(* Logix 5000 Routine export JVL_MAC2; software revision 37.00 *)

TYPE JVL_AXIS_MAC_G3 :   // Drive Data
STRUCT
   ActualMode : DINT;   // actual Mode
   ActualPosition : REAL;   // P_IST
   ActualVelocity : REAL;   // V_IST(16)
   ActualTorque : REAL;   // ACTUAL_TORQUE
   AxisStatusError : JVL_MAC_Status_Error;   // Holds an indication of which error that is detected
   Home_Mode : DINT;   // Homemode
   RequestedMode : DINT;   // requested Mode
   RequestedPosition : REAL;   // P_SOLL
   RequestedVelocity : REAL;   // V_SOLL
   RequestedAcceleration : REAL;   // A_SOLL
   GeneralCommand : DINT;
   CommandTorque : REAL;   // Requested Torque, T_SOLL
   ZeroSearchVelocity : REAL;   // Homing velocity
   ZeroSearchPosition : REAL;   // Homing position
   ZeroSearchTorque : DINT;   // Homing torque setpoint threshold value
   ZeroSearchTThreshold : DINT;   // Threshold for torque zerosearch trigger, usually 20% lower than running torque
   TravelConst : REAL;   // Factor to multiply P_IST and P_SOLL for scaling
   VelConst : REAL;   // Factor to multiply V_SOLL and V_IST to get scaled velocity value
   HomingType : DINT;   // Holds the reqested homingtype
   LoadFactor : DINT;   // Inertia ratio motor/load
   MotorType : DINT;   // MotorType configured. 0=No Selection 1=MAC50-141-A/K (old) 2=MAC50-141-F (new), MAC400, 402, 1500, 3000, 4500 (All Encoder variations) 3=MAC800 with incremental encoder 4=MAC800 with abs. encoder
   Configured : DINT;
   MSG_OutValue : DINT;   // Used in exp. output message to the motor
   MSG_InValue : DINT;   // Used in Exp. output message, to get value from motor
   MSG_OutInstance : DINT;   // Registernumber
   MSG_InInstance : DINT;   // Registernummer
   V_SOLL_CountsPerSample : REAL;
   A_SOLL_CountsPerSample2 : REAL;
   AOI_Type : DINT;   // MAC_Disable = 1, MAC_Home = 2, MAC_Jog = 3, MAC_Position = 4, MAC_Reset = 5, MAC_Stop = 6
   Position_AppType : REAL;   // calculated Position by Application Type
   MSG_Out_Execute : BOOL;   // Enable MSG_Out
   MSG_In_Execute : BOOL;   // Enable MSG_In
   ErrorReset : BOOL;
   MSG_Out_Busy : BOOL;
   MSG_In_Busy : BOOL;
   MSG_Out_Done : BOOL;
   MSG_In_Done : BOOL;
END_STRUCT
END_TYPE

TYPE JVL_MAC_Status_Error :   // Axis Faults Status
STRUCT
   Error : BOOL;
   InitialisationError : BOOL;
   FlashMemoryError : BOOL;
   STOError : BOOL;
   NotUsed_2 : BOOL;
   NotUsed_3 : BOOL;
   OUT1 : BOOL;
   OUT2 : BOOL;
   NotUsed : BOOL;
   ControlVoltageError : BOOL;
   HomingDone : BOOL;
   MotorSupplyDetected : BOOL;
   MotorLocked : BOOL;
   CommsError : BOOL;
   CurrentLoopError : BOOL;
   ModbusSlaveError : BOOL;
   TemperatureError : BOOL;
   UndervoltageError : BOOL;
   UndervoltageDetect : BOOL;
   OvervoltageError : BOOL;
   OvercurrentError : BOOL;
   OverspeedError : BOOL;
   AllowExceedingOfSoftwareLimits : BOOL;
   EncoderError : BOOL;
   I2TError : BOOL;
   FollowingError : BOOL;
   FunctionError : BOOL;
   BreakingResistorOverTempError : BOOL;
   InPosition : BOOL;
   Accelerating : BOOL;
   Decelerating : BOOL;
   SoftwareLimitExceeded : BOOL;
END_STRUCT
END_TYPE

ADD_ON_INSTRUCTION MAC_G3_COM   (* revision 1.0 *)
VAR_IN_OUT
   JVL_IN : _03A8:MACG3Servomotor_939149E5:I:0; {required}
   JVL_OUT : _03A8:MACG3Servomotor_D07D4DE6:O:0; {required}
   MSG_IN : MESSAGE; {required}
   MSG_OUT : MESSAGE; {required}
   AXIS : JVL_AXIS_MAC_G3; {required}
END_VAR
VAR_INPUT
   ApplicationType : DINT; {required}   // Application_Type - 0=none (counts) 1=linear 2=degree
   TravelPerRev : REAL := 1.0; {required}   // Travel per Revolution. Exc. actuator w. 60mm/rev, then value=60
   GearRatio : REAL := 1.0; {required}   // Gear ratio if a gearbox is mounted. select 1 for none
   RequestedTorque : DINT := 100; {required}   // Torque in %, 0-300%
   MotorType : DINT;   // 0=MAC_G3 1=MAC50-141-A/K (old) 2=MAC50-141-F (new), MAC400, 402, 1500, 3000, 4500 (All Encoder variations) 3=MAC800 with incremental encoder 4=MAC800 with abs. encoder
END_VAR
VAR
   CountsPerRevolution : REAL; {access None}
   vel : INT; {access None}
   torque : INT; {access None}
END_VAR

ROUTINE Logic   (* structured text *)
   
   
   	//MAC050F-141F (new mini MAC), MAC400, MAC402, MAC1500-MAC4500
   	IF MotorType = 2 THEN
   	    AXIS.V_SOLL_CountsPerSample := 2.84;
   	    AXIS.A_SOLL_CountsPerSample2 := 0.003693;
   		CountsPerRevolution:= 8192.0;
   	//MAC800-MAC1200 incremental encoder
   	ELSIF MotorType = 3 THEN
   	    AXIS.V_SOLL_CountsPerSample := 2.77;
   	    AXIS.A_SOLL_CountsPerSample2 := 0.003606;
   		CountsPerRevolution:= 8000.0;
   	//MAC800-MAC1200 absolute encoder
   	ELSIF MotorType = 4 THEN
   	    AXIS.V_SOLL_CountsPerSample := 2.84;
   	    AXIS.A_SOLL_CountsPerSample2 := 0.003606;
   		CountsPerRevolution:= 8192.0;
   	//new MAC G3
   	ELSIF MotorType = 0 THEN
   	    AXIS.V_SOLL_CountsPerSample := 2.133;
   	    AXIS.A_SOLL_CountsPerSample2 := 0.002133;
   		CountsPerRevolution:= 8192.0;
   	//MAC050-141-A/K (old mini MAC)
   	ELSIF MotorType = 1 THEN
   	    AXIS.V_SOLL_CountsPerSample := 2.1;
   	    AXIS.A_SOLL_CountsPerSample2 := 0.004026;
   		CountsPerRevolution:= 4096.0;
   	ELSE
   	    AXIS.V_SOLL_CountsPerSample := 0.0;
   	    AXIS.A_SOLL_CountsPerSample2 := 0.0;
   	END_IF;
   
   	AXIS.MotorType := MotorType;
   
   	//counts
   	if ApplicationType = 0 then
   	AXIS.TravelConst := 1;
   	AXIS.VelConst:= AXIS.V_SOLL_CountsPerSample;
   	//linear
   	elsif ApplicationType = 1 then
   	AXIS.TravelConst :=(CountsPerRevolution * GearRatio) / TravelPerRev;
   	AXIS.VelConst:= AXIS.V_SOLL_CountsPerSample * 60 * GearRatio / TravelPerRev;
   	//360°
   	elsif ApplicationType = 2 then
   	AXIS.TravelConst :=(CountsPerRevolution * GearRatio) / 360;
   	AXIS.VelConst:= AXIS.V_SOLL_CountsPerSample * 60 * GearRatio / 360;
   	end_if;
   
   
   AXIS.ActualMode := JVL_IN.Operation_Mode;
   AXIS.ActualPosition := JVL_IN.Actual_Position;
   //AXIS.ActualVelocity := JVL_IN.Data[2];
   //AXIS.ActualTorque := JVL_IN.Data[3];
   vel:=JVL_IN.Actual_Velocity;
   torque:=JVL_IN.Actual_Torque;
   if MotorType=1 then
   
   AXIS.ActualVelocity := trunc(vel*7.63);
   AXIS.ActualTorque := trunc(torque * 0.293);
   else
   AXIS.ActualVelocity := trunc(vel/AXIS.VelConst);
   AXIS.ActualTorque := trunc(torque * 0.293);
   end_if;
   //AXIS.Home_Mode := JVL_IN.Data[5];
   
   AXIS.Position_AppType:= (AXIS.ActualPosition/AXIS.TravelConst);
   AXIS.AxisStatusError.Error := JVL_IN.An_Error_is_present;
   AXIS.AxisStatusError.InitialisationError := JVL_IN.Internal_Initialization_Error;
   AXIS.AxisStatusError.FlashMemoryError := JVL_IN.Flash_Memory_Error;
   AXIS.AxisStatusError.STOError := JVL_IN.STO_Circuitry_Error;
   //AXIS.AxisStatusError.NotUsed_2 := JVL_IN.Data[4].28;
   //AXIS.AxisStatusError.NotUsed_3 := JVL_IN.Data[4].29;
   //AXIS.AxisStatusError.OUT1 := JVL_IN.Data[4].30;
   //AXIS.AxisStatusError.OUT2 := JVL_IN.Data[4].31;
   //AXIS.AxisStatusError.NotUsed := JVL_IN.Data[4].16;
   AXIS.AxisStatusError.ControlVoltageError := JVL_IN.Unstable_Controlvoltage_24V;
   AXIS.AxisStatusError.HomingDone := JVL_IN.Error_And_Status.18;
   AXIS.AxisStatusError.MotorSupplyDetected := JVL_IN.AC_Voltage_Present;
   AXIS.AxisStatusError.MotorLocked := JVL_IN.PWM_Locked_Critical_Error;
   AXIS.AxisStatusError.CommsError := JVL_IN.Error_And_Status.21;
   AXIS.AxisStatusError.CurrentLoopError := JVL_IN.Error_And_Status.22;
   AXIS.AxisStatusError.ModbusSlaveError := JVL_IN.Error_And_Status.23;
   AXIS.AxisStatusError.TemperatureError := JVL_IN.Temperature_Error;
   AXIS.AxisStatusError.UndervoltageError := JVL_IN.Undervoltage_Error1;
   AXIS.AxisStatusError.UndervoltageDetect := JVL_IN.Undervoltage_Error2;
   AXIS.AxisStatusError.OvervoltageError := JVL_IN.Overvoltage_Error;
   AXIS.AxisStatusError.OvercurrentError := JVL_IN.Error_And_Status.12;
   AXIS.AxisStatusError.OverspeedError := JVL_IN.Overspeed_Error;
   AXIS.AxisStatusError.AllowExceedingOfSoftwareLimits := JVL_IN.Position_Limit_Disabled;
   AXIS.AxisStatusError.EncoderError := JVL_IN.Internal_Encoder_Error;
   AXIS.AxisStatusError.I2TError := JVL_IN.I2T_Overload_Error;
   AXIS.AxisStatusError.FollowingError := JVL_IN.Follow_Error;
   AXIS.AxisStatusError.FunctionError := JVL_IN.Function_error;
   AXIS.AxisStatusError.BreakingResistorOverTempError := JVL_IN.Error_And_Status.3;
   AXIS.AxisStatusError.InPosition := JVL_IN.In_Position;
   AXIS.AxisStatusError.Accelerating := JVL_IN.Accelerating;
   AXIS.AxisStatusError.Decelerating := JVL_IN.Decelerating;
   AXIS.AxisStatusError.SoftwareLimitExceeded := JVL_IN.Position_Limit_Error;
   
   JVL_OUT.Operation_Mode:= AXIS.RequestedMode;
   //cop(AXIS.RequestedPosition,JVL_OUT.Data[1],4);
   JVL_OUT.Requested_Position:= AXIS.RequestedPosition;
   //cop(AXIS.RequestedVelocity,JVL_OUT.Data[2],4);
   JVL_OUT.Target_Velocity:= AXIS.RequestedVelocity;
   JVL_OUT.Target_Acceleration:= AXIS.RequestedAcceleration;
   JVL_OUT.General_Command:= AXIS.GeneralCommand;
   AXIS.CommandTorque:=RequestedTorque*3.41;
   JVL_OUT.Target_Torque:=AXIS.CommandTorque;
   AXIS.MSG_Out_Done:= MSG_OUT.DN;
   AXIS.MSG_Out_Busy:= MSG_OUT.EN;
   AXIS.MSG_In_Done:= MSG_IN.DN;
   AXIS.MSG_In_Busy:= MSG_IN.EN;
   
   MSG_OUT.Instance:= AXIS.MSG_OutInstance;
   MSG_IN.Instance:= AXIS.MSG_InInstance;
   
END_ROUTINE
END_ADD_ON_INSTRUCTION

ADD_ON_INSTRUCTION MAC_G3_MAFR   (* revision 1.0, ExecuteEnableInFalse *)
VAR_IN_OUT
   AXIS : JVL_AXIS_MAC_G3; {required}
END_VAR
VAR_OUTPUT
   EN : BOOL; {access Read Only, visible}
   CommandAborted : BOOL; {access Read Only}
   DN : BOOL; {access Read Only, visible}
   ER : BOOL; {visible}
END_VAR
VAR
   State : INT; {access None}
   ExecuteStart : BOOL; {access None}
   AOI_Type : DINT; {access None}
END_VAR

ROUTINE EnableInFalse   (* structured text *)
   State := 0;
   ExecuteStart:=0;
   	//REGION STATUS SIGNALS
   
   	    DN := State = 30;
   	    CommandAborted := State = 80;
   	    EN := EnableOut;
   	    ER:= AXIS.AxisStatusError.Error;
   	//END_REGION
   
END_ROUTINE

ROUTINE Logic   (* structured text *)
   	(*********************
   		Error Reset
   	**********************)
   
   	//REGION CAPTURE EDGES
   	    if EnableIn and not ExecuteStart then
   	    	ExecuteStart:=1;
   		//elsif not EnableIn then
   			//ExecuteStart:=0;
   		end_if;
   
   	//END_REGION
   
   	//REGION STATE CHANGES
   
   	    //Re-trigger sequence from start on rising edge
   	    //Command aborted
   	    IF AXIS.AOI_Type <> AOI_Type AND
   	        State <> 0 AND
   	        State <> 90 AND
   	        State <> 30 AND
   	        State <> 80
   	    THEN
   	        State := 80;
   	    END_IF;
   
   
   	//END_REGION
   
   	//REGION STATE MACHINE
   
   	    CASE State OF
   
   	        0:
   	            IF ExecuteStart THEN
   					AOI_Type:= 5;
   					AXIS.AOI_Type:= 5;
   	                AXIS.GeneralCommand := 16#0;
   	                State := 10;
   	            END_IF;
   
   	        10:
   	            AXIS.RequestedMode := 0;
   	            AXIS.RequestedAcceleration := 0;
   	            AXIS.RequestedPosition := 0;
   	            AXIS.RequestedVelocity := 0;
   	            AXIS.GeneralCommand := 16#10000E1;
   	            IF NOT AXIS.AxisStatusError.Error and AXIS.MotorType<>1 THEN
   	                State := 20;
   
   	            END_IF;
   
   
   	        20:
   	            AXIS.GeneralCommand := 16#0;
   	            State := 30;
   
   	        30:        //reset complete, reset to idle by setting execute false
   	            ;
   
   	        80:     //Aborted by other command before completion
   	            ;
   
   	        90:       //Error while disabling, reset to idle by setting execute false
   	            ;
   
   	        ELSE
   	            ;
   
   	    END_CASE;
   
   	//END_REGION
   
   	//REGION STATUS SIGNALS
   
   	    DN := State = 30;
   	    CommandAborted := State = 80;
   	    EN := EnableOut;
   	    ER:= AXIS.AxisStatusError.Error;
   	//END_REGION
   
END_ROUTINE
END_ADD_ON_INSTRUCTION

ADD_ON_INSTRUCTION MAC_G3_MAH   (* revision 1.0, ExecuteEnableInFalse *)
VAR_IN_OUT
   Axis : JVL_AXIS_MAC_G3; {required}
END_VAR
VAR_OUTPUT
   CommandAborted : BOOL; {access Read Only}
   EN : BOOL; {access Read Only, visible}   // Enable Bit - The EN bit stays Set until the Process is Complete and the rung goes False
   DN : BOOL; {access Read Only, visible}   // Done Bit - The Done bit is Set if the Instruction Executed without Errors
   ER : BOOL; {access Read Only, visible}   // Error Bit - An Error Happened
   IP : BOOL; {access Read Only, visible}   // In Progress Bit - The In Progress bit is Set While the Axis is Moving
   PC : BOOL; {access Read Only, visible}   // Process Complete, Motion has stopped
END_VAR
VAR_INPUT
   Mode : INT; {required}   // 0 = set Encoder, 1 = Homing on Sensor, 2 = Homing on Block
   Position : REAL; {required}   // Scaled Position after setting Encoder, with Mode = 0
   Speed : REAL; {required}   // Scaled velocity
   Acceleration : REAL; {required}   // in RPM/s
   Offset : REAL; {required}   // scaled Position after Homing, with Mode = 1 or 2
   TorqueLimit : REAL; {required}   // Homing Torque in %
END_VAR
VAR
   State : INT; {access None}
   ActiveMode : INT; {access None}
   Mode0State : INT; {access None}
   Mode1State : INT; {access None}
   Mode2State : INT; {access None}
   Mode3State : INT; {access None}
   ActivePosition : DINT; {access None}
   ActiveVelocity : DINT; {access None}
   ActiveAcceleration : REAL; {access None}
   ActiveTorqueLimit : REAL; {access None}
   ExecuteStart : BOOL; {access None}
   AOI_Type : DINT; {access None}
   ActiveDeceleration : DINT; {access None}
   Ton_wait : FBD_TIMER; {access None}
   ActiveOffset : DINT; {access None}
END_VAR

ROUTINE EnableInFalse   (* structured text *)
   State := 0;
   ExecuteStart:=0;
   	//REGION STATUS SIGNALS
   
   	    DN := State = 30;
   	    CommandAborted := State = 80;
   	    ER := State = 90;
   	    IP := State <> 0 AND NOT DN AND NOT ER AND NOT CommandAborted;
   	    EN := EnableOut;
   		PC := State = 30;
   	//END_REGION
END_ROUTINE

ROUTINE Logic   (* structured text *)
   	//REGION CAPTURE EDGES
   	    if EnableIn and not ExecuteStart then
   	    	ExecuteStart:=1;
               Axis.MSG_Out_Execute := 0;
               Axis.MSG_In_Execute := 0;
   			Ton_wait.TimerEnable:=0;
   			Ton_wait.Reset:=0;
   		elsif not EnableIn then
   			ExecuteStart:=0;
   		end_if;
   
   	//END_REGION
   	//Timer
   	TONR(Ton_wait);
   
   	//REGION STATE CHANGES
   
   	    //Re-trigger sequence from start on rising edge
   
   
   	    //Command aborted
   	    IF Axis.AOI_Type <> AOI_Type AND
   	        State <> 0 AND
   	        State <> 90 AND
   	        State <> 30 AND
   	        State <> 80
   	    THEN
   	        State := 80;
   	    END_IF;
   
   
   	    //Error if motor error while executing
   	    IF Axis.AxisStatusError.Error AND
   	        State <> 0 AND
   	        State <> 90 AND
   	        State <> 30 AND
   	        State <> 80
   	    THEN
   	        State := 90;
   	    END_IF;
   	//END_REGION
   
   	//REGION STATE MACHINE
   
   
   
   	    CASE State OF
   
   	        0:
   	            //Reset static values
   	            ActiveMode := 0;
   	            ActivePosition := 0;
   	            ActiveVelocity := 0;
   				ActiveAcceleration := 0;
   	            ActiveDeceleration := 0;
   				ActiveTorqueLimit := 0;
   	            ActiveOffset := 0;
   	            //Reset mode states
   	            Mode0State := 0;
   	            Mode1State := 0;
   	            Mode2State := 0;
   	            Mode3State := 0;
   
   	            IF ExecuteStart THEN
   					//
   					AOI_Type:= 2;
   					Axis.AOI_Type:= 2;
   	                //
   					Axis.GeneralCommand := 0;
   	                ActiveMode := Mode;
   	                ActivePosition := Position * Axis.TravelConst;
   	                ActiveVelocity := (Speed) * Axis.VelConst;// * Axis.Device.Config.V_SOLL_CountsPerSample);
   	                ActiveAcceleration := ABS(Acceleration) * Axis.A_SOLL_CountsPerSample2;
   	                //set Acceleration always >=1
   	                IF ActiveAcceleration < 1 THEN
   	                    ActiveAcceleration := 1;
   	                END_IF;
   
   	                ActiveTorqueLimit := TorqueLimit * 3.41;//1024=300%;341=100%
   	                ActiveOffset := Offset * Axis.TravelConst;
   
   
   	                State := 10;
   	            END_IF;
   
   	        10:
   	            // change to velocity mode with zero setpoint to ensure motor does not run off to current position when homed
   	            IF ActiveAcceleration < 1 THEN
   	                Axis.RequestedAcceleration := 1;
   	            ELSE
   	                Axis.RequestedAcceleration := ActiveAcceleration;
   
   	            END_IF;
   	            Axis.RequestedVelocity := 0;
   	            Axis.RequestedMode := 1;
   	            // change position setpoint to new home position
   	            Axis.RequestedPosition := ActivePosition;
   	            // reset register trigger
   	            Axis.MSG_Out_Execute := 0;
   	            Axis.MSG_In_Execute := 0;
   	            // start homing
   	            State := 20;
   
   	        20:
   	            CASE ActiveMode OF
   
   	                0:  // Set Home Position
   	                    CASE Mode0State OF
   	                        0:
   	                            if Axis.MotorType=1 then
   									Axis.MSG_OutInstance := 163;
   								else
   									Axis.MSG_OutInstance := 4;
   								end_if;
   	                            Axis.MSG_OutValue:=ActivePosition;
   	                            Axis.MSG_Out_Execute := 1;
   	                            Axis.GeneralCommand := 16#0;
   	                            IF Axis.MSG_Out_Busy AND NOT Axis.MSG_Out_Done THEN
   	                                Mode0State := 10;
   	                            END_IF;
   	                        10:
   	                            IF Axis.MSG_Out_Done THEN
   	                                Axis.MSG_Out_Execute := 0;
   	                                Mode0State := 20;
   	                            END_IF;
   	                        20:
   	                            Axis.GeneralCommand := 16#10000F7;
   	                            IF ABS(Axis.ActualPosition - ActivePosition) < 50.0 THEN
   	                                Mode0State := 30;
   	                            END_IF;
   	                        30:
   	                            Axis.GeneralCommand := 16#0;
   	                            Mode0State := 50;
   	                        50:
   	                            State := 30;
   	                        ELSE
   	                            State := 90;
   	                    END_CASE;
   
   	                1:  // Home to Sensor (type 2, bidirectional)
   	                    CASE Mode1State OF
   	                       0:
   	                            // reset hominging done bit old MAC050-141A/K
   	                                IF Axis.MotorType <> 1 THEN
   	                                    Mode1State := 10;
   	                                ELSE
   		                            Axis.MSG_OutInstance := 168;
   		                            Axis.MSG_OutValue := 0;
   		                            Axis.MSG_Out_Execute := 1;
   			                            IF Axis.MSG_Out_Busy THEN
   			                                Mode1State := 5;
   			                            END_IF;
   	                                END_IF;
   	                        5:
   	                            //Ton_Wait(IN := Reg.Done,PT := t#1s);
   	                            IF Axis.MSG_Out_Done THEN
   	                                Axis.MSG_Out_Execute := 0;
   	                                Mode1State := 10;
   	                            END_IF;
   	                       10:
   	                            //Home to Sensor (type 2);set homemode=3584
   	                            Axis.MSG_OutInstance := 42;
   	                            Axis.MSG_OutValue:=3584;
   
   	                            Axis.MSG_Out_Execute := 1;
   	                            IF Axis.MSG_Out_Busy THEN
   	                                Mode1State := 15;
   	                            END_IF;
   	                       15:
   	                            IF Axis.MSG_Out_Done THEN
   	                                Axis.MSG_Out_Execute := 0;
   	                                Mode1State := 20;
   									Axis.AxisStatusError.HomingDone:=0;
   	                            END_IF;
   
   	                       20:
   	                            // set home position offset move distance
   	                            Axis.MSG_OutInstance := 38;
   	                            Axis.MSG_OutValue:=ActiveOffset;
   	                            Axis.MSG_Out_Execute := 1;
   	                            IF Axis.MSG_Out_Busy THEN
   	                                Mode1State := 30;
   	                            END_IF;
   	                        30:
   	                            IF Axis.MSG_Out_Done THEN
   	                                Axis.MSG_Out_Execute := 0;
   	                                Mode1State := 40;
   	                            END_IF;
   	                        40:
   	                            // set homing approach velocity
   	                            Axis.MSG_OutInstance := 40;
   	                            Axis.MSG_OutValue:=ActiveVelocity;// * Axis.Device.Config.V_SOLL_CountsPerSample
   	                            Axis.MSG_Out_Execute := 1;
   	                            IF Axis.MSG_Out_Busy THEN
   	                                Mode1State := 50;
   	                            END_IF;
   	                        50:
   	                            IF Axis.MSG_Out_Done THEN
   	                                Axis.MSG_Out_Execute := 0;
   	                                Mode1State := 60;
   	                            END_IF;
   	                        60:
   	                            // start homing mode
   	                            Axis.RequestedMode := 14;
   								if Axis.MotorType=1 then
   									Axis.RequestedVelocity := ActiveVelocity;
   								end_if;
   	                            if Axis.ActualMode=14 then
   	                            	Mode1State := 70;
   	                            end_if;
   	                        70:
   	                            IF Axis.AxisStatusError.HomingDone AND Axis.MotorType <> 1 THEN
   	                                Axis.RequestedVelocity := 0;
   	                                Axis.RequestedMode := 2;
   	                                Mode1State := 80;
   	                            ELSIF Axis.Home_Mode > 0 AND Axis.MotorType = 1 THEN
   	                                Axis.RequestedVelocity := 0;
   	                                Axis.RequestedMode := 2;
   	                                Mode1State := 80;
   	                            END_IF;
   	                        80:
   	                            State := 30;
   	                        ELSE
   	                            State := 90;
   	                    END_CASE;
   
   	                2:  // Home to Endstop (torque limit)
   	                    CASE Mode2State OF
   	                        0:
   	                            //Home to Endstop (torque limit);set homemode=3072
   								Axis.MSG_OutInstance := 42;
   	                            Axis.MSG_OutValue := 3072;
   	                            Axis.MSG_Out_Execute := 1;
   
   	                            IF Axis.MSG_Out_Busy THEN
   	                                Mode2State := 5;
   	                            END_IF;
   	                        5:
   	                            IF Axis.MSG_Out_Done THEN
   	                                Axis.MSG_Out_Execute := 0;
   	                                Mode2State := 10;
   	                            END_IF;
   	                        10:
   								Axis.MSG_OutInstance := 38;
   	                            Axis.MSG_OutValue := ActiveOffset;
   	                            Axis.MSG_Out_Execute := 1;
   
   	                            IF Axis.MSG_Out_Busy THEN
   	                                Mode2State := 15;
   	                            END_IF;
   	                        15:
   	                            IF Axis.MSG_Out_Done THEN
   	                                Axis.MSG_Out_Execute := 0;
   	                                Mode2State := 20;
   									Axis.AxisStatusError.HomingDone:=0;
   	                            END_IF;
   	                        20:
   								Axis.MSG_OutInstance := 40;
   	                            Axis.MSG_OutValue := ActiveVelocity;// * Axis.Device.Config.V_SOLL_CountsPerSample;
   	                            Axis.MSG_Out_Execute := 1;
   	                            IF Axis.MSG_Out_Busy THEN
   	                                Mode2State := 25;
   	                            END_IF;
   	                        25:
   	                            IF Axis.MSG_Out_Done THEN
   	                                Axis.MSG_Out_Execute := 0;
   	                                IF Axis.MotorType <> 1 THEN
   	                                    Mode2State := 34;
   	                                ELSE
   	                                    Mode2State := 30;
   	                                END_IF;
   	                            END_IF;
   	                        30:
   	                            // reset hominging done bit old MAC050-141A/K
   								Axis.MSG_OutInstance := 168;
   	                            Axis.MSG_OutValue := 0;
   	                            Axis.MSG_Out_Execute := 1;
   
   	                            IF Axis.MSG_Out_Busy THEN
   	                                Mode2State := 32;
   	                            END_IF;
   	                        32:
   
   	                            IF Axis.MSG_Out_Done THEN
   	                                Axis.MSG_Out_Execute := 0;
   	                                Mode2State := 34;
   	                            END_IF;
   	                        34:
   								Axis.MSG_OutInstance := 41;
   	                            Axis.MSG_OutValue := ActiveTorqueLimit;
   	                            Axis.MSG_Out_Execute := 1;
   
   	                            IF Axis.MSG_Out_Busy THEN
   	                                Mode2State := 37;
   	                            END_IF;
   	                        37:
   	                            IF Axis.MSG_Out_Done THEN
   	                                Axis.MSG_Out_Execute := 0;
   	                                Mode2State := 40;
   	                            END_IF;
   	                        40:
   	                            Axis.RequestedMode := 12;
   	                            // homing done-register 42 Homemode bit 16
   								if Axis.MotorType=1 then
   									Axis.RequestedVelocity := ActiveVelocity;
   								end_if;
   	                            if Axis.ActualMode=12 then
   	                            	Mode2State := 45;
   	                            end_if;
   
   	                        45:
   	                            IF Axis.AxisStatusError.HomingDone AND Axis.MotorType <> 1 THEN
   	                                Axis.RequestedVelocity := 0;
   	                                Axis.RequestedMode := 2;
   	                                Mode2State := 60;
   	                            ELSIF Axis.Home_Mode > 0 AND Axis.MotorType = 1 THEN
   	                                Axis.RequestedVelocity := 0;
   	                                Axis.RequestedMode := 2;
   	                                Mode2State := 60;
   	                            END_IF;
   
   	                        60:
   	                            State := 30;
   	                        ELSE
   	                            State := 90;
   	                    END_CASE;
   
   
   
   	            END_CASE;
   
   	        30:        //Home complete, reset to idle by setting execute false
   	            ;
   
   	        80:     //Aborted by other command before completion
   	            ;
   
   	        90:       //Error while disabling, reset to idle by setting execute false
   	            ;
   
   	        ELSE
   	            ;
   
   	    END_CASE;
   
   	//END_REGION
   
   	//REGION STATUS SIGNALS
   
   	    DN := State = 30;
   	    CommandAborted := State = 80;
   	    ER := State = 90;
   	    IP := State <> 0 AND NOT DN AND NOT ER AND NOT CommandAborted;
   	    EN := EnableOut;
   		PC := State = 30;
   	//END_REGION
END_ROUTINE
END_ADD_ON_INSTRUCTION

ADD_ON_INSTRUCTION MAC_G3_MAJ   (* revision 1.0, ExecuteEnableInFalse *)
VAR_IN_OUT
   AXIS : JVL_AXIS_MAC_G3; {required}
END_VAR
VAR_INPUT
   Direction : DINT; {required}   // 0 = CW rotation, 1 = CCW rotation
   Speed : REAL; {required}   // scaled velocity
   Acceleration : REAL := 5000.0; {required}   // in rpm/s
END_VAR
VAR_OUTPUT
   EN : BOOL; {access Read Only, visible}   // Enable Bit - The EN bit stays Set until the Process is Complete and the rung goes False
   DN : BOOL; {access Read Only, visible}   // Done Bit - The Done bit is Set if the Instruction Executed without Errors
   ER : BOOL; {access Read Only, visible}   // Error Bit - An Error Happened
   IP : BOOL; {access Read Only, visible}   // In Progress Bit - The In Progress bit is Set While the Axis is Moving
END_VAR
VAR
   ForwardStart : BOOL; {access None}
   BackwardStart : BOOL; {access None}
   State : INT; {access None}
   ActiveVelocity : REAL; {access None}
   ActiveAcceleration : REAL; {access None}
   AOI_Type : DINT; {access None}
   ActiveDeceleration : REAL; {access None}
END_VAR

ROUTINE EnableInFalse   (* structured text *)
   	//REGION CAPTURE EDGES
   	    if Direction = 0 and EnableIn then
   	    	ForwardStart:=1;
   	    elsif Direction = 1 and EnableIn then
   	    	BackwardStart:=1;
   		elsif not EnableIn then
   	    	ForwardStart:=0;
   	    	BackwardStart:=0;
   		end_if;
   
   	//END_REGION
   
   	//REGION STATE CHANGES
   
   	    //Re-trigger sequence from start on rising edge
   	    //Command aborted
   	    IF AXIS.AOI_Type <> AOI_Type AND
   	        State <> 0 AND
   	        State <> 90 AND
   	        State <> 80
   	    THEN
   	        State := 80;
   	    END_IF;
   
   
   
   	    //Error if motor error while executing
   	    IF AXIS.AxisStatusError.Error AND
   	        State <> 0 AND
   	        State <> 90 AND
   	        State <> 80
   	    THEN
   	        State := 90;
   	    END_IF;
   
   	//END_REGION
   
   	//REGION STATE MACHINE
   
   	    CASE State OF
   
   	        0:
   	            ActiveVelocity := 0;
   	            ActiveAcceleration := 0;
   	            ActiveDeceleration := 0;
   
   	            IF ForwardStart OR BackwardStart THEN
   					DN := 0;
   					AOI_Type:= 3;
   					AXIS.AOI_Type:= 3;
   	                AXIS.RequestedMode:= 1;
   	                ActiveAcceleration := ABS(Acceleration);
   
   	                //set Acceleration always >=1
   	                IF ActiveAcceleration < 1 THEN
   	                    ActiveAcceleration := 1;
   	                END_IF;
   	                IF Direction = 0 THEN
   	                    ActiveVelocity := ABS(Speed) * AXIS.VelConst;// * Axis.Device.Config.V_SOLL_CountsPerSample));
   	                    State := 10;
   	                ELSIF Direction = 1 THEN
   	                    ActiveVelocity := -1.0 * ABS(Speed)* AXIS.VelConst;// * Axis.Device.Config.V_SOLL_CountsPerSample));
   	                    State := 10;
   	                ELSE
   	                    State := 30;
   	                END_IF;
   
   	                State := 10;
   	            END_IF;
   
   	        10:
   	            IF AXIS.ActualMode = 1 THEN
   
   	                AXIS.RequestedAcceleration := ActiveAcceleration;
   	                AXIS.RequestedVelocity := ActiveVelocity;
                       State := 30;
   
   	            END_IF;
   
   	        20:
   	            IF AXIS.ActualMode = 1 THEN
   
   	                IF not EnableIn THEN
   	                    State := 30;
   	                END_IF;
   
   	            ELSE
   	                State := 80;
   	            END_IF;
   
   
   	        30:
   	            AXIS.RequestedMode := 1;
   	            AXIS.RequestedVelocity := 0;
   
   	            State := 40;
   
   	        40:
   	            IF AXIS.ActualMode = 1  THEN
   
   	                //If no motion then stop is complete
   	                IF ABS((AXIS.ActualVelocity)) <= 10.0 AND
   	                    NOT AXIS.AxisStatusError.Accelerating AND
   	                    NOT AXIS.AxisStatusError.Decelerating THEN
   	                    State := 0;
   						DN := 1;
   	                END_IF;
   
   	            ELSE
   	                State := 80;
   	            END_IF;
   
   	        80:     //Aborted by other command before completion
   	            IF NOT EnableIn THEN
   	                State := 0;
   	            END_IF;
   
   	        90:       //Error while jogging, reset to idle by setting jog inputs false
   	            IF NOT EnableIn THEN
   	                State := 0;
   	            END_IF;
   
   	        ELSE
   	            State := 90;
   
   	    END_CASE;
   
   	//END_REGION
   
   	//REGION STATUS SIGNALS
   
   	    EN:=EnableOut;
   						//(State=20 or State = 25) AND
   	                    //  AXIS.AxisStatus.AtVelocity AND
   	                    //  NOT AXIS.AxisStatus.Accelerating AND
   	                    //  NOT AXIS.AxisStatus.Decelerating;
   	    DN := State = 40;
   	    ER := State = 90;
   	    IP := State <> 0 AND NOT ER AND NOT DN;
   
   	//END_REGION
   
END_ROUTINE

ROUTINE Logic   (* structured text *)
   	//REGION CAPTURE EDGES
   	    if Direction = 0 and EnableIn then
   	    	ForwardStart:=1;
   	    elsif Direction = 1 and EnableIn then
   	    	BackwardStart:=1;
   		elsif not EnableIn then
   	    	ForwardStart:=0;
   	    	BackwardStart:=0;
   		end_if;
   
   	//END_REGION
   
   	//REGION STATE CHANGES
   
   	    //Re-trigger sequence from start on rising edge
   	    //Command aborted
   	    IF AXIS.AOI_Type <> AOI_Type AND
   	        State <> 0 AND
   	        State <> 90 AND
   	        State <> 80
   	    THEN
   	        State := 80;
   	    END_IF;
   
   
   
   	    //Error if motor error while executing
   	    IF AXIS.AxisStatusError.Error AND
   	        State <> 0 AND
   	        State <> 90 AND
   	        State <> 80
   	    THEN
   	        State := 90;
   	    END_IF;
   
   	//END_REGION
   
   	//REGION STATE MACHINE
   
   	    CASE State OF
   
   	        0:
   	            ActiveVelocity := 0;
   	            ActiveAcceleration := 0;
   	            ActiveDeceleration := 0;
   
   	            IF ForwardStart OR BackwardStart THEN
   					DN := 0;
   					AOI_Type:= 3;
   					AXIS.AOI_Type:= 3;
   	                AXIS.RequestedMode:= 1;
   	                ActiveAcceleration := ABS(Acceleration)* AXIS.A_SOLL_CountsPerSample2;
   	                //set Acceleration always >=1
   	                IF ActiveAcceleration < 1 THEN
   	                    ActiveAcceleration := 1;
   	                END_IF;
   	                IF Direction = 0 THEN
   	                    ActiveVelocity := ABS(Speed) * AXIS.VelConst;// * Axis.Device.Config.V_SOLL_CountsPerSample));
   	                    State := 10;
   	                ELSIF Direction = 1 THEN
   	                    ActiveVelocity := -1.0 * ABS(Speed)* AXIS.VelConst;// * Axis.Device.Config.V_SOLL_CountsPerSample));
   	                    State := 10;
   	                ELSE
   	                    State := 30;
   	                END_IF;
   
   	                State := 10;
   	            END_IF;
   
   	        10:
   	            IF AXIS.ActualMode = 1 THEN
   
   	                AXIS.RequestedAcceleration := ActiveAcceleration;
   	                AXIS.RequestedVelocity := ActiveVelocity;
   	                IF not EnableIn THEN
   	                    State := 30;
   	                END_IF;
   
   	            END_IF;
   
   	        20:
   	            IF AXIS.ActualMode = 1 THEN
   
   	                IF not EnableIn THEN
   	                    State := 30;
   	                END_IF;
   
   	            ELSE
   	                State := 80;
   	            END_IF;
   
   
   	        30:
   	            AXIS.RequestedMode := 1;
   	            AXIS.RequestedVelocity := 0;
   
   	            State := 40;
   
   	        40:
   	            IF AXIS.ActualMode = 1  THEN
   
   	                //If no motion then stop is complete
   	                IF ABS((AXIS.ActualVelocity)) <= 10.0 AND
   	                    NOT AXIS.AxisStatusError.Accelerating AND
   	                    NOT AXIS.AxisStatusError.Decelerating THEN
   	                    State := 0;
   						DN := 1;
   	                END_IF;
   
   	            ELSE
   	                State := 80;
   	            END_IF;
   
   	        80:     //Aborted by other command before completion
   	            IF NOT EnableIn THEN
   	                State := 0;
   	            END_IF;
   
   	        90:       //Error while jogging, reset to idle by setting jog inputs false
   	            IF NOT EnableIn THEN
   	                State := 0;
   	            END_IF;
   
   	        ELSE
   	            State := 90;
   
   	    END_CASE;
   
   	//END_REGION
   
   	//REGION STATUS SIGNALS
   
   	    EN:=EnableOut;
   						//(State=20 or State = 25) AND
   	                    //  AXIS.AxisStatus.AtVelocity AND
   	                    //  NOT AXIS.AxisStatus.Accelerating AND
   	                    //  NOT AXIS.AxisStatus.Decelerating;
   	    DN := State = 40;
   	    ER := State = 90;
   	    IP := State <> 0 AND NOT ER AND NOT DN;
   
   	//END_REGION
   
END_ROUTINE
END_ADD_ON_INSTRUCTION

ADD_ON_INSTRUCTION MAC_G3_MAM   (* revision 1.0, ExecuteEnableInFalse *)
VAR_IN_OUT
   Axis : JVL_AXIS_MAC_G3; {required}
END_VAR
VAR_INPUT
   MoveType : DINT; {required}   // 0=absolute, 1= relative
   Position : REAL; {required}   // scaled Position
   Speed : REAL; {required}   // scaled velocity
   Acceleration : REAL; {required}   // in rpm/s
END_VAR
VAR_OUTPUT
   CommandAborted : BOOL; {access Read Only}
   EN : BOOL; {visible}   // Enable Bit - The EN bit stays Set until the Process is Complete and the rung goes False
   DN : BOOL; {access Read Only, visible}   // Done Bit - The Done bit is Set if the Instruction Executed without Errors
   ER : BOOL; {access Read Only, visible}   // Error Bit - An Error Happened
   IP : BOOL; {access Read Only, visible}   // In Progress Bit - The In Progress bit is Set While the Axis is Moving
   PC : BOOL; {visible}   // Process Complete, Motion has stopped
END_VAR
VAR
   State : INT; {access None}
   ExecuteStart : BOOL; {access None}
   ActiveAbsolute : BOOL; {access None}
   ActiveVelocity : DINT; {access None}
   ActiveAcceleration : REAL; {access None}
   ActiveTargetPosition : DINT; {access None}
   StartPosition : REAL; {access None}
   AOI_Type : DINT; {access None}
END_VAR

ROUTINE EnableInFalse   (* structured text *)
   State := 0;
   ExecuteStart:=0;
   	    DN := State = 30 OR State = 35;
   		PC:= State = 30 OR State = 35;
   	    CommandAborted := State = 80;
   	    ER := State = 90;
   	    IP := State <> 0 AND NOT DN AND NOT ER AND NOT CommandAborted;
   	    EN:= EnableOut;
   
END_ROUTINE

ROUTINE Logic   (* structured text *)
   	//REGION CAPTURE EDGES
   	    if EnableIn and not ExecuteStart then
   	    	ExecuteStart:=1;
   			State:= 0;
   
   		end_if;
   
   	//END_REGION
   
   	//REGION STATE CHANGES
   
   	    //Re-trigger sequence from start on rising edge
   
   
   	    //Command aborted
   	    IF Axis.AOI_Type <> AOI_Type AND
   	        State <> 0 AND
   	        State <> 90 AND
   	        State <> 30 AND
   	        State <> 80
   	    THEN
   	        State := 80;
   	    END_IF;
   
   
   	    //Error if motor error while executing
   	    IF Axis.AxisStatusError.Error AND
   	        State <> 0 AND
   	        State <> 90 AND
   	        State <> 30 AND
   	        State <> 80
   	    THEN
   	        State := 90;
   	    END_IF;
   	//END_REGION
   
   	//REGION STATE MACHINE
   
   	    CASE State OF
   
   	        0:
   	            ActiveVelocity := 0;
   	            ActiveAcceleration := 0;
   				ActiveAbsolute := 0;
   	            ActiveTargetPosition := 0;
   
   	            IF ExecuteStart THEN
   					AOI_Type:= 4;
   					Axis.AOI_Type:= 4;
   	                Axis.RequestedMode := 2;
   	                StartPosition := Axis.ActualPosition;// *Axis.TravelConst;
   	                ActiveVelocity := ABS(Speed) * Axis.VelConst;// * Axis.Device.Config.V_SOLL_CountsPerSample);
   	                ActiveAcceleration := ABS(Acceleration)* Axis.A_SOLL_CountsPerSample2;
   	                //set Acceleration always >=1
   	                IF ActiveAcceleration < 1.0 THEN
   	                    ActiveAcceleration := 1.0;
   	                END_IF;
   
   					if MoveType= 0 then
   	                	ActiveAbsolute := 1;
   					elsif MoveType = 1 then
   						ActiveAbsolute:= 0;
   					end_if;
   
   
   
   	                IF ActiveAbsolute THEN
   	                    ActiveTargetPosition := Position *Axis.TravelConst;
   	                ELSE
   	                    ActiveTargetPosition := Position *Axis.TravelConst+ StartPosition;
   	                END_IF;
   
   	                State := 10;
   	            END_IF;
   
   	        10:
   	            IF Axis.ActualMode = 2 THEN
   	                Axis.RequestedAcceleration := ActiveAcceleration;
   	                Axis.RequestedPosition := ActiveTargetPosition;
   	                Axis.RequestedVelocity := ActiveVelocity;
   
   					State := 20;
   					(*
   	                IF ContinuousUpdate THEN
   	                    State := 25;
   	                ELSE
   	                    State := 20;
   	                END_IF;
   	                *)
   	            END_IF;
   
   	        20:
   	            IF Axis.ActualMode = 2 AND
   	                Axis.RequestedPosition = ActiveTargetPosition AND
   	                Axis.RequestedVelocity = ActiveVelocity THEN
   
   	                //If taget reached then move is complete
   	                IF ABS(ActiveTargetPosition - Axis.ActualPosition) <= 10 AND
   	                    Axis.AxisStatusError.InPosition AND
   	                    NOT Axis.AxisStatusError.Accelerating AND
   	                    NOT Axis.AxisStatusError.Decelerating THEN
   	                    State := 30;
   	                END_IF;
   
   	            ELSE
   	                State := 80;
   	            END_IF;
   
   	        30:
   	            ;
   	        (*
   	        25:
   	            IF Axis.Telegram.Input.OperatingMode = 2 AND
   	                Axis.Telegram.Output.VelocitySetpoint = DINT_TO_DWORD(ActiveVelocity) AND
   	                Axis.Telegram.Output.PositionSetpoint = DINT_TO_DWORD(ActiveTargetPosition) THEN
   
   	                IF Execute THEN
   
   	                    ActiveVelocity := LREAL_TO_DINT(ABS(Velocity) * Axis.Device.Config.V_SOLL_CountsPerSample);
   	                    ActiveAcceleration := LREAL_TO_DINT(ABS(Acceleration) * Axis.Device.Config.A_SOLL_CountsPerSample2);
   	                    //set Acceleration always >=1
   	                    IF ActiveAcceleration < 1 THEN
   	                        ActiveAcceleration := 1;
   	                    END_IF;
   	                    IF ActiveAbsolute THEN
   	                        ActiveTargetPosition := Position;
   	                    ELSE
   	                        ActiveTargetPosition := Position + StartPosition;
   	                    END_IF;
   
   	                    Axis.Telegram.Output.AccelerationSetpoint := ActiveAcceleration;
   	                    Axis.Telegram.Output.PositionSetpoint := ActiveTargetPosition;
   	                    Axis.Telegram.Output.VelocitySetpoint := ActiveVelocity;
   
   	                    //If taget reached then move is complete
   	                    IF ABS(DINT_TO_LREAL(ActiveTargetPosition - Axis.Telegram.Input.ActualPosition)) <= 5.0 AND
   	                        Axis.Telegram.Input.StatusError.InPosition AND
   	                        NOT Axis.Telegram.Input.StatusError.Accelerating AND
   	                        NOT Axis.Telegram.Input.StatusError.Decelerating THEN
   	                        State := 35;
   	                    END_IF;
   
   	                ELSE
   	                    State := 20;
   	                END_IF;
   
   	            ELSE
   	                State := 80;
   	            END_IF;
   
   	        35:
   	            IF Execute THEN
   
   	                IF ActiveAbsolute THEN
   	                    IF ActiveTargetPosition <> Position THEN
   	                        State := 20;
   	                    END_IF;
   	                ELSE
   	                    IF ActiveTargetPosition <> (Position + StartPosition) THEN
   	                        State := 25;
   	                    END_IF;
   	                END_IF;
   
   	            ELSE
   	                State := 0;
   	            END_IF;
   	        *)
   	        80:     //Aborted by other command before completion
   	           ;
   
   	        90:       //Error, reset to idle by setting execute false
   	            ;
   	            //Mode=Passiv
   	            Axis.RequestedMode := 0;
   	        ELSE
   	            ;
   
   	    END_CASE;
   
   	//END_REGION
   
   	//REGION STATUS SIGNALS
   
   	    DN := State = 30 OR State = 35;
   		PC:= State = 30 OR State = 35;
   	    CommandAborted := State = 80;
   	    ER := State = 90;
   	    IP := State <> 0 AND NOT DN AND NOT ER AND NOT CommandAborted;
   	    EN:= EnableOut;
   	//END_REGION
END_ROUTINE
END_ADD_ON_INSTRUCTION

ADD_ON_INSTRUCTION MAC_G3_MAS   (* revision 1.0, ExecuteEnableInFalse *)
VAR_IN_OUT
   AXIS : JVL_AXIS_MAC_G3; {required}
END_VAR
VAR_INPUT
   Decel_Rate : REAL; {required}   // in RPM/s
END_VAR
VAR_OUTPUT
   CommandAborted : BOOL; {access Read Only}
   EN : BOOL; {access Read Only, visible}
   DN : BOOL; {access Read Only, visible}
   ER : BOOL; {access Read Only, visible}
   IP : BOOL; {access Read Only, visible}
   PC : BOOL; {access Read Only, visible}
END_VAR
VAR
   State : INT; {access None}
   ExecuteStart : BOOL; {access None}
   ActiveDeceleration : DINT; {access None}
   AOI_Type : DINT; {access None}
END_VAR

ROUTINE EnableInFalse   (* structured text *)
   State := 0;
   ExecuteStart:=0;
   
   	    DN := State = 30;
   	    CommandAborted := State = 80;
   	    ER := State = 90;
   	    IP := State<> 0 AND NOT DN AND NOT ER AND NOT CommandAborted;
   	    EN:=EnableOut;
   		PC := State = 30;
   
END_ROUTINE

ROUTINE Logic   (* structured text *)
   	//REGION CAPTURE EDGES
   	    if EnableIn and not ExecuteStart then
   	    	ExecuteStart:=1;
   
   		end_if;
   
   	//END_REGION
   
   	//REGION STATE CHANGES
   
   	    //Re-trigger sequence from start on rising edge
   
   	    //Command aborted
   	    IF AXIS.AOI_Type <> AOI_Type AND
   	        State <> 0 AND
   	        State <> 90 AND
   	        State <> 30 AND
   	        State <> 80
   	    THEN
   	        State := 80;
   	    END_IF;
   
   	    //Error if motor error while executing
   	    IF AXIS.AxisStatusError.Error AND
   	        State <> 0 AND
   	        State <> 90 AND
   	        State <> 30 AND
   	        State <> 80
   	    THEN
   	        State := 90;
   	    END_IF;
   
   	//END_REGION
   
   	//REGION STATE MACHINE
   
   	    CASE State OF
   
   	        0:        //Wait for rising edge on execute
   	            ActiveDeceleration := 0;
   
   	            IF ExecuteStart THEN
   					AOI_Type:= 6;
   					AXIS.AOI_Type:= 6;
   	                AXIS.RequestedMode:= 1;
   	                ActiveDeceleration :=  Decel_Rate;//
   	                //set Acceleration always >=1
   	                IF ActiveDeceleration < 1 THEN
   	                    ActiveDeceleration := 1;
   	                END_IF;
   	                State := 10;
   	            END_IF;
   
   	        10:        //Trigger stop
   	            IF AXIS.ActualMode = 1 THEN
   	                AXIS.RequestedAcceleration := ActiveDeceleration;
   	                AXIS.RequestedVelocity := 0;
   	                State := 20;
   
   	            ELSE            //Go to Idle if other command has changed the operating state
   	                State := 0;
   	            END_IF;
   
   	        20:    //Check stop is complete
   	            IF AXIS.RequestedMode = 1 AND
   	                AXIS.RequestedVelocity = 0 THEN
   
   	                //If no motion then stop is complete
   	                IF ABS(AXIS.ActualVelocity) <= 10.0 AND
   	                    NOT AXIS.AxisStatusError.Accelerating and
   	                    NOT AXIS.AxisStatusError.Decelerating THEN
   	                    State := 30;
   	                END_IF;
   
   	            ELSE            //Go to Idle if other command has changed the operating state
   	                State := 0;
   	            END_IF;
   
   	        30:        //Disable complete, reset to idle by setting execute false
   	            IF NOT EnableIn THEN
   	                ;
   	            END_IF;
   
   	        80:     //Aborted by other command before completion
   	            IF NOT EnableIn THEN
   					;
   				END_IF;
   
   	        90:       //Error while disabling, reset to idle by setting execute false
   	            IF NOT EnableIn THEN
   	                ;
   	            END_IF;
   
   	        ELSE
   	            ;
   
   	    END_CASE;
   
   	//END_REGION
   
   	//REGION STATUS SIGNALS
   
   	    DN := State = 30;
   	    CommandAborted := State = 80;
   	    ER := State = 90;
   	    IP := State<> 0 AND NOT DN AND NOT ER AND NOT CommandAborted;
   	    EN:=EnableOut;
   		PC := State = 30;
   
   	//END_REGION
END_ROUTINE
END_ADD_ON_INSTRUCTION

ADD_ON_INSTRUCTION MAC_G3_MSF   (* revision 1.0, ExecuteEnableInFalse *)
VAR_IN_OUT
   AXIS : JVL_AXIS_MAC_G3; {required}
END_VAR
VAR_OUTPUT
   EN : BOOL; {access Read Only, visible}
   CommandAborted : BOOL; {access Read Only}
   DN : BOOL; {access Read Only, visible}
   ER : BOOL; {access Read Only, visible}
END_VAR
VAR
   State : INT; {access None}
   ExecuteStart : BOOL; {access None}
   AOI_Type : DINT; {access None}
END_VAR

ROUTINE EnableInFalse   (* structured text *)
   State := 0;
   ExecuteStart:=0;
   	//REGION STATUS SIGNALS
   
   	    DN := State = 20;
   	    CommandAborted := State = 80;
   	    ER := State = 90;
   	    EN := EnableOut;
   
   	//END_REGION
   
END_ROUTINE

ROUTINE Logic   (* structured text *)
   	///REGION CAPTURE EDGES
   
   	 	if EnableIn and not ExecuteStart then
   	    	ExecuteStart:=1;
   		end_if;
   	///END_REGION
   
   	//REGION STATE CHANGES
   
   	    //Re-trigger sequence from start on rising edge
   
   	    //Command aborted
   	    IF AXIS.AOI_Type <> AOI_Type AND
   	        State <> 0 AND
   	        State <> 90 AND
   	        State <> 30 AND
   	        State <> 80
   	    THEN
   	        State := 80;
   	    END_IF;
   
   
   	    //Error if motor error while executing
   	    IF AXIS.AxisStatusError.Error AND
   	        State <> 0 AND
   	        State <> 90 AND
   	        State <> 20 AND
   	        State <> 80
   	    THEN
   	        State := 90;
   	    END_IF;
   
   	//END_REGION
   
   	//REGION STATE MACHINE
   
   	    CASE State OF
   
   	        0:        //Wait for rising edge on execute
   	            IF ExecuteStart THEN
   					AOI_Type:= 1;
   					AXIS.AOI_Type:= 1;
   	                State := 10;
   	            END_IF;
   
   	        10:     //Put JVL into passive state
   	            AXIS.RequestedMode:= 0;
   	            IF AXIS.ActualMode = 0 THEN
   	                State := 20;
   	            END_IF;
   
   	        20:        //Disable complete, reset to idle by setting execute false
   	            ;
   
   	        80:     //Aborted by other command before completion
   	            ;
   
   	        90:       //Error while disabling, reset to idle by setting execute false
   	           ;
   
   	        ELSE
   	            ;//State := 90;
   
   	    END_CASE;
   
   	//END_REGION
   
   	//REGION STATUS SIGNALS
   
   	    DN := State = 20;
   	    CommandAborted := State = 80;
   	    ER := State = 90;
   	    EN := EnableOut;
   
   	//END_REGION
   
END_ROUTINE
END_ADD_ON_INSTRUCTION

VAR_GLOBAL   (* controller tags *)
   M1 : DINT;
   M1_Disable : MAC_G3_MSF;
   M1_Home : MAC_G3_MAH := (Mode := 1, Position := 100.0, Speed := 10.0, Acceleration := 5000.0, Offset := 10.0, TorqueLimit := 17.0);
   M1_Jog : MAC_G3_MAJ := (Speed := 50.0, Acceleration := 5000.0);
   M1_Position : MAC_G3_MAM := (Speed := 100.0, Acceleration := 5000.0);
   M1_Reset : MAC_G3_MAFR;
   M1_Stop : MAC_G3_MAS;
   M1Axis : JVL_AXIS_MAC_G3 := (ActualPosition := 368790.0, AxisStatusError.HomingDone := 1, AxisStatusError.MotorSupplyDetected := 1, AxisStatusError.AllowExceedingOfSoftwareLimits := 1, RequestedAcceleration := 10.665, CommandTorque := 341.0, TravelConst := 819.2, VelConst := 12.797999, MSG_OutValue := 128, MSG_OutInstance := 40, V_SOLL_CountsPerSample := 2.133, A_SOLL_CountsPerSample2 := 0.002133, AOI_Type := 1, Position_AppType := 450.1831, MSG_Out_Done := 1);
   M1com : MAC_G3_COM := (ApplicationType := 1, TravelPerRev := 10.0, GearRatio := 1.0, RequestedTorque := 100);
   MSG_M1In : MESSAGE;
        MessageParameters(MessageType := CIP Generic, ConnectedFlag := 2, ConnectionPath := M1, ServiceCode := 16#000e, ObjectType := 16#0064, AttributeNumber := 16#0001, DestinationTag := M1Axis.MSG_InValue)
   MSG_M1Out : MESSAGE;
        MessageParameters(MessageType := CIP Generic, RequestedLength := 4, ConnectedFlag := 2, ConnectionPath := M1, ServiceCode := 16#0010, ObjectType := 16#0064, TargetObject := 40, AttributeNumber := 16#0001, LocalElement := M1Axis.MSG_OutValue)
END_VAR

PROGRAM MainProgram
VAR
   TonIn : TIMER := (PRE := 50);
   TonOut : TIMER := (PRE := 50);
END_VAR

ROUTINE JVL_MAC2   (* ladder *)
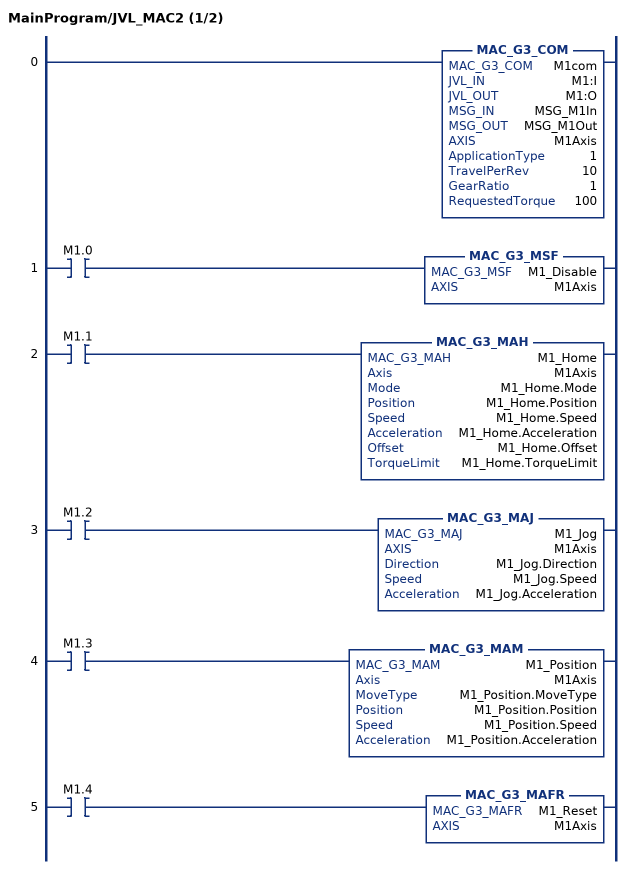
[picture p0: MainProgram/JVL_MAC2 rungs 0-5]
   0: MAC_G3_COM(M1com,M1:I,M1:O,MSG_M1In,MSG_M1Out,M1Axis,1,10,1,100);
   1: XIC(M1.0)MAC_G3_MSF(M1_Disable,M1Axis);
   2: XIC(M1.1)MAC_G3_MAH(M1_Home,M1Axis,M1_Home.Mode,M1_Home.Position,M1_Home.Speed,M1_Home.Acceleration,M1_Home.Offset,M1_Home.TorqueLimit);
   3: XIC(M1.2)MAC_G3_MAJ(M1_Jog,M1Axis,M1_Jog.Direction,M1_Jog.Speed,M1_Jog.Acceleration);
   4: XIC(M1.3)MAC_G3_MAM(M1_Position,M1Axis,M1_Position.MoveType,M1_Position.Position,M1_Position.Speed,M1_Position.Acceleration);
   5: XIC(M1.4)MAC_G3_MAFR(M1_Reset,M1Axis);
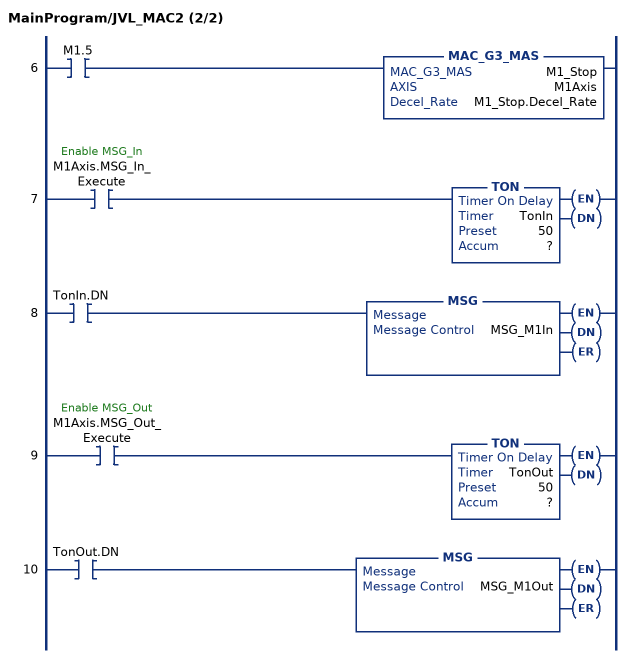
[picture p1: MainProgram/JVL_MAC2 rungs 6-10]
   6: XIC(M1.5)MAC_G3_MAS(M1_Stop,M1Axis,M1_Stop.Decel_Rate);
   7: XIC(M1Axis.MSG_In_Execute)TON(TonIn,?,?);
   8: XIC(TonIn.DN)MSG(MSG_M1In);
   9: XIC(M1Axis.MSG_Out_Execute)TON(TonOut,?,?);
   10: XIC(TonOut.DN)MSG(MSG_M1Out);
END_ROUTINE
END_PROGRAM
